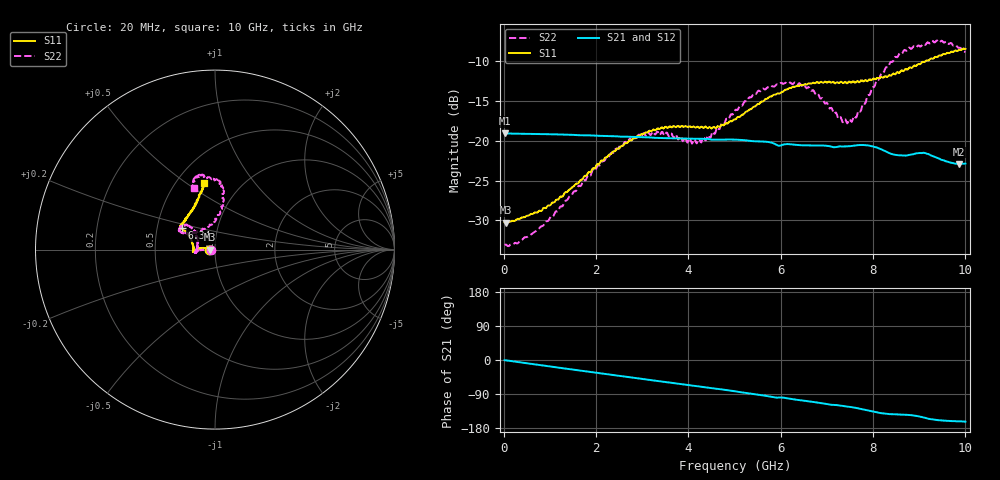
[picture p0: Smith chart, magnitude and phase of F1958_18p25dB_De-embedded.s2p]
! Integrated Device Technology
! Corporate Headquarters
! 6024 Silver Creek Valley Road
! San Jose, CA 95138  USA
! Phone:  1-408-284-8200
! Toll Free:  1-800-223-1366
! Webpage:  http://www.idt.com/
! Timing and RF Division
! 515 Groton Road, Suite 102
! Westford, MA 01886-6024
! Device:  F1958
! Description: 7-bit 0.25 dB Digital Step Attenuator
! Frequency:  0.001 -  6.000 GHz
! Package:  4x4 mm Thin QFN Plastic Package: 24 pin
! Ports:  2 RF, 12 DC
!  Pin  1  = D0
!  Pin  2  = VDD
!  Pin  3  = VMODE
!  Pin  4  = GND
!  Pin  5  = RF1  =  Port 1
!  Pin  6  = GND
!  Pin  7  = GND
!  Pin  8  = GND
!  Pin  9  = GND
!  Pin 10  = GND
!  Pin 11  = GND
!  Pin 12  = GND
!  Pin 13  = GND
!  Pin 14  = RF2  =  Port 2
!  Pin 15  = GND
!  Pin 16  = LE
!  Pin 17  = CLK
!  Pin 18  = DATA
!  Pin 19  = D6
!  Pin 20  = D5
!  Pin 21  = D4
!  Pin 22  = D3
!  Pin 23  = D2
!  Pin 24  = D1
! State:  73
! Atten State:  18.25 dB
! Voltage:  +3.30 Volts
! Current:  0.258 mA
! Data:  The device was measured on a F1958 evaluation board which has
!  individual transmission lines to the RF pins.  Data was collected
!  using a calibrated network analyzer.  The evaluation board was
!  de-embedded using Automatic Fixture Removal (AFR).
!  The reference plane is the edge of the package pin.
! Misc:
!  Action Tracker AT0419
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# GHz S dB R 50
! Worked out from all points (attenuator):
!   500 points, 20 MHz to 10 GHz, reference 50 ohm
!   highest |S21| = -19.07 dB at 20 MHz (marker M1); lowest = -22.9 dB at 9.86 GHz (marker M2)
!   lowest |S11| = -30.3 dB at 40 MHz (marker M3), VSWR 1.06, Z = 47 - j0.0462 ohm
!   |S11| at or under -10 dB: start of sweep to 9.136 GHz
!   |S22| runs from -33.2 to -7.4 dB; largest |S21 - S12| = 0.00045
!   S11 on the Smith chart (normalised r, x): 20 MHz: 0.94, -0.00; 6.34 GHz: 0.67, +0.17; 10 GHz: 0.68, +0.59
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0.02  -30.25 -178.9  -19.07 -0.4  -19.07 -0.4  -33.09 -178.0
0.04  -30.29 -179.1  -19.08 -0.8  -19.07 -0.7  -33.03 -177.1
0.32  -29.81 175.4  -19.11 -5.6  -19.11 -5.5  -32.80 179.1
0.72  -29.03 173.1  -19.15 -12.3  -19.15 -12.3  -31.24 -179.7
1.7  -24.88 171.8  -19.31 -28.5  -19.30 -28.5  -25.28 179.8
2.6  -20.55 177.6  -19.48 -43.3  -19.46 -43.4  -20.38 -176.6
2.92  -19.39 -178.7  -19.53 -48.6  -19.52 -48.7  -19.25 -173.7
3.36  -18.52 -175.2  -19.64 -55.9  -19.64 -56.0  -19.14 -170.0
4.24  -18.39 -178.8  -19.75 -69.9  -19.76 -70.0  -19.81 167.4
4.5  -18.46 175.4  -19.85 -74.6  -19.86 -74.6  -19.21 151.9
5.02  -17.32 160.9  -19.86 -82.8  -19.86 -82.8  -16.11 138.3
5.56  -15.21 150.5  -20.08 -92.2  -20.10 -92.2  -13.79 138.9
6.34  -13.12 147.6  -20.51 -104.9  -20.53 -104.9  -12.92 151.8
6.68  -12.75 146.3  -20.58 -110.2  -20.60 -110.1  -13.69 151.7
7.3  -12.58 140.6  -20.71 -120.5  -20.71 -120.3  -17.03 129.6
7.48  -12.56 137.4  -20.68 -123.5  -20.68 -123.4  -17.34 111.3
7.68  -12.57 135.0  -20.54 -127.5  -20.54 -127.5  -16.27 94.5
8.34  -11.78 118.9  -21.52 -142.7  -21.51 -142.7  -10.60 80.4
8.68  -11.13 112.1  -21.86 -144.4  -21.87 -144.4  -8.59 85.2
9.26  -9.66 104.4  -21.86 -156.3  -21.87 -156.4  -7.57 98.4
9.86  -8.61 99.5  -22.91 -161.8  -22.96 -161.7  -8.33 107.7
10  -8.47 99.5  -22.86 -162.9  -22.90 -162.7  -8.88 108.5
